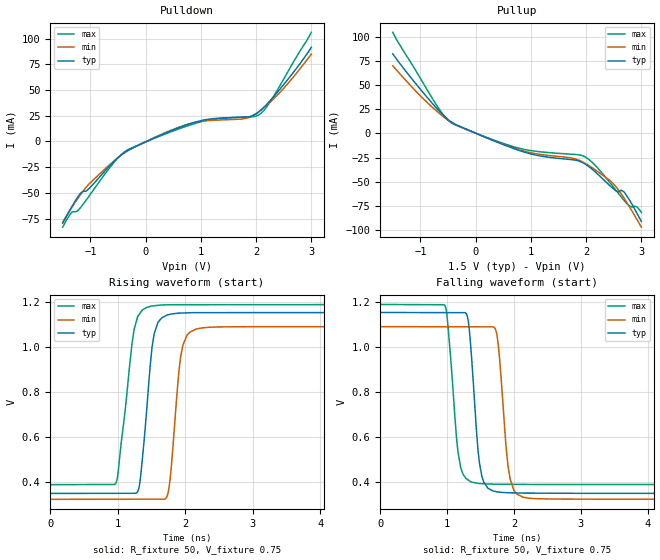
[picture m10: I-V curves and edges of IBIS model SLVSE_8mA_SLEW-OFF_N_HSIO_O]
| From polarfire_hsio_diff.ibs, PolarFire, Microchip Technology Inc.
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|   Model SLVSE_8mA_SLEW-OFF_N_HSIO_O
[Model]   SLVSE_8mA_SLEW-OFF_N_HSIO_O
Model_type   Output
Polarity   Inverting
Enable   Active-High
Vmeas =   0.2
Cref =   5p
Rref =   100
|   typ   min   max
C_comp_pullup   1.335e-12   1.335e-12   1.380e-12
C_comp_pulldown  1.335e-12   1.335e-12   1.380e-12
[Temperature Range]  25C   100C   -40C
[Voltage Range]  1.5   1.425   1.575
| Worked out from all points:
|   slope of the pulldown table from 0 to 0.225 V, typ, clamps not added: 41.3 ohm
|   slope of the pullup table from 0 to 0.225 V, typ, clamps not added: 41.3 ohm
|   rising waveform, R_fixture 50, V_fixture 0.75: 20-80 % time 139ps typ, 128ps min, 177ps max; typ from 0.35 V to 1.15 V
|   falling waveform, R_fixture 50, V_fixture 0.75: 20-80 % time 118ps typ, 121ps min, 126ps max; typ from 1.15 V to 0.35 V
[Pulldown]
| Voltage   I(typ)   I(min)   I(max)
-1.5V     -79.31mA   -78.36mA   -83.19mA
-1.329V   -62.78mA   -63.64mA   -68.27mA
-1.181V   -50.43mA   -51.83mA   -64.44mA
-1.034V   -46.25mA   -41.83mA   -53.81mA
-590.6mV  -20.36mA   -19.68mA   -21.52mA
-344.5mV  -9.397mA   -9.826mA   -8.704mA
750mV     16.29mA    16.47mA    15.01mA
1.219V    22.12mA    20.56mA    21.62mA
1.845V    23.91mA    22.78mA    23.84mA
2.091V    30.58mA    30.69mA    27.43mA
2.484V    54.25mA    50.76mA    59.11mA
3V        91.37mA    84.77mA    106mA
[Pullup]
| Voltage   I(typ)   I(min)   I(max)
-1.5V     82.17mA    69.83mA    104.3mA
-689.1mV  25.02mA    22.3mA     27.64mA
-443mV    11.95mA    11.6mA     11.09mA
796.9mV   -17.71mA   -16.94mA   -15.39mA
1.697V    -26.83mA   -24.95mA   -21.3mA
1.943V    -30.31mA   -29.56mA   -23.13mA
2.189V    -40.87mA   -38.59mA   -34.37mA
2.534V    -58.98mA   -54.43mA   -58.14mA
2.681V    -60.01mA   -66.29mA   -68.66mA
2.78V     -68.2mA    -75.24mA   -74.76mA
2.927V    -83.06mA   -89.5mA    -75.97mA
3V        -90.94mA   -96.74mA   -81.58mA
[Ramp]
dV/dt_r   0.481251/0.13889n  0.459325/0.12837n  0.479027/0.176635n
dV/dt_f   0.481268/0.117679n  0.459346/0.121135n  0.479048/0.12572n
R_load = 50
[Rising Waveform]
R_fixture = 50
V_fixture = 0.75
V_fixture_min = 0.7125
V_fixture_max = 0.7875
| Time   V(typ)   V(min)   V(max)
0s        350mV      323.8mV    388.9mV
976ps     350.5mV    324.3mV    397.9mV
1.209ns   350.6mV    324.5mV    1.008V
1.293ns   356.8mV    324.5mV    1.131V
1.352ns   462.7mV    324.5mV    1.157V
1.501ns   975mV      324.6mV    1.18V
1.749ns   1.142V     355.7mV    1.186V
1.931ns   1.149V     952.3mV    1.186V
2.159ns   1.151V     1.078V     1.186V
10ns      1.152V     1.089V     1.187V
[Falling Waveform]
R_fixture = 50
V_fixture = 0.75
V_fixture_min = 0.7125
V_fixture_max = 0.7875
| Time   V(typ)   V(min)   V(max)
0s        1.152V     1.09V      1.188V
968ps     1.152V     1.089V     1.182V
1.161ns   1.152V     1.089V     535.3mV
1.315ns   1.117V     1.089V     409.5mV
1.408ns   762.7mV    1.089V     397.5mV
1.519ns   425.5mV    1.089V     393.5mV
1.725ns   358.7mV    1.076V     391.2mV
1.909ns   353.3mV    472.7mV    390.7mV
2.134ns   351.8mV    333.4mV    390.3mV
10ns      350.3mV    324.1mV    389.4mV
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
